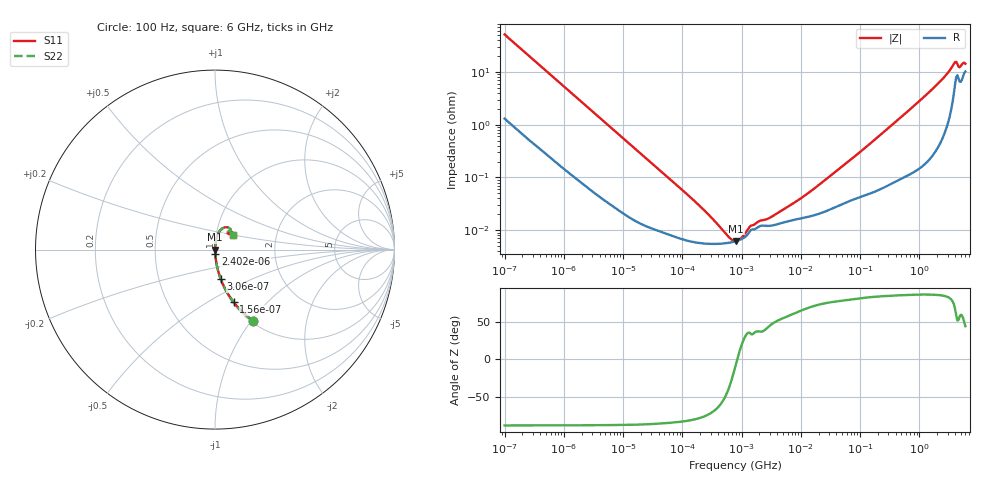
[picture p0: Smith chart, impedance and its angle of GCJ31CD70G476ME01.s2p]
!Murata Part Number: GCJ31CD70G476ME01
!These Parameters are Measured in Series Mode Connection
!Data Generated on Mar 13, 2026
!  o--ll--o
!Port1  Port2
!  o------o
!Operation Temp=25[degC], DC Bias Voltage=0[V]
!Freq. Start=100[Hz] Stop=6[GHz] 401[Steps]
# Hz S RI R 50
!Freq.(Hz) S11(Real) S11(Imag) S21(Real) S21(Imag) S12(Real) S12(Imag) S22(Real) S22(Imag)
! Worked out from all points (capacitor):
!   401 points, 100 Hz to 6 GHz, reference 50 ohm
!   read as one part in series: C = 30.9 uF near 109 Hz
!   lowest |Z| = 6.25 mohm at 810.1 kHz (marker M1)
!   series resonance near 844.2 kHz, so ESL is about 1.2 nH
!   S11 on the Smith chart (normalised r, x): 100 Hz: 1.03, -1.03; 156 Hz: 1.02, -0.66; 306 Hz: 1.01, -0.34; 2.402 kHz: 1.00, -0.04; 6 GHz: 1.20, +0.20
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100  0.214 -0.3976  0.786 0.3976  0.786 0.3976  0.214 -0.3976
156  0.1043 -0.2933  0.8957 0.2933  0.8957 0.2933  0.1043 -0.2933
306  0.0322 -0.1642  0.9678 0.1642  0.9678 0.1642  0.0322 -0.1642
717  0.00737 -0.0732  0.9926 0.0732  0.9926 0.0732  0.00737 -0.0732
2008  0.0015 -0.0268  0.9985 0.0268  0.9985 0.0268  0.0015 -0.0268
2402  0.00117 -0.0225  0.9988 0.0225  0.9988 0.0225  0.00117 -0.0225
40335  9.83e-05 -0.00141  0.9999 0.00141  0.9999 0.00141  9.83e-05 -0.00141
184852  5.78e-05 -0.000303  0.9999 0.000303  0.9999 0.000303  5.78e-05 -0.000303
452617  5.57e-05 -9.29e-05  0.9999 9.29e-05  0.9999 9.29e-05  5.57e-05 -9.29e-05
517687  5.65e-05 -7.11e-05  0.9999 7.11e-05  0.9999 7.11e-05  5.65e-05 -7.11e-05
774597  6.13e-05 -1.21e-05  0.9999 1.21e-05  0.9999 1.21e-05  6.13e-05 -1.21e-05
810067  6.22e-05 -5.8e-06  0.9999 5.8e-06  0.9999 5.8e-06  6.22e-05 -5.8e-06
1159002  7.55e-05 4.57e-05  0.9999 -4.57e-05  0.9999 -4.57e-05  7.55e-05 4.57e-05
1983483  0.000118 9.06e-05  0.9999 -9.06e-05  0.9999 -9.06e-05  0.000118 9.06e-05
2967816  0.000121 0.000121  0.9999 -0.000121  0.9999 -0.000121  0.000121 0.000121
1.555665e7  0.000188 0.000545  0.9998 -0.000545  0.9998 -0.000545  0.000188 0.000545
3.124326e8  0.000805 0.00893  0.9992 -0.00893  0.9992 -0.00893  0.000805 0.00893
1.791126e9  0.00546 0.0507  0.9945 -0.0507  0.9945 -0.0507  0.00546 0.0507
3.065283e9  0.0199 0.0939  0.9801 -0.0939  0.9801 -0.0939  0.0199 0.0939
3.8344e9  0.0542 0.1241  0.9458 -0.1241  0.9458 -0.1241  0.0542 0.1241
4.796499e9  0.0706 0.0902  0.9294 -0.0902  0.9294 -0.0902  0.0706 0.0902
6e9  0.0999 0.0819  0.9001 -0.0819  0.9001 -0.0819  0.0999 0.0819
